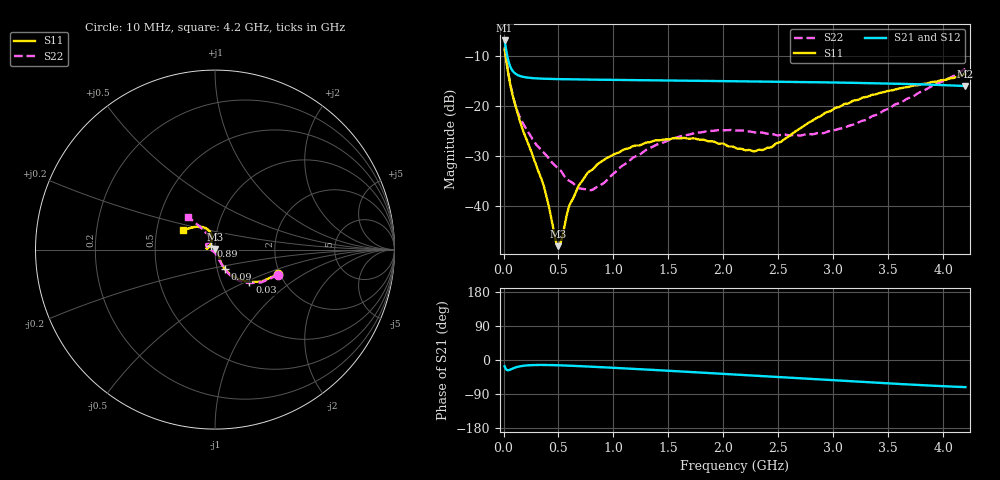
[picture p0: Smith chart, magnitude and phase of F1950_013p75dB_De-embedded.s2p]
! Integrated Device Technology
! Corporate Headquarters
! 6024 Silver Creek Valley Road
! San Jose, CA 95138  USA
! Phone:  1-408-284-8200
! Toll Free:  1-800-223-1366
! Webpage:  http://www.idt.com/
! Timing and RF Division
! 515 Groton Road, Suite 102
! Westford, MA 01886-6024
! Device:  F1950
! Description: 7-bit 0.25 dB Digital Step Attenuator
! Frequency:  150.0 -  4000.00 MHz
! Package:  4x4 mm Thin QFN Plastic Package: 24 pin
! Ports:  2 RF, 12 DC
!  Pin  1  = D0
!  Pin  2  = VDD
!  Pin  3  = Vmode
!  Pin  4  = GND
!  Pin  5  = RF1  =  Port 1
!  Pin  6  = GND
!  Pin  7  = GND
!  Pin  8  = GND
!  Pin  9  = GND
!  Pin 10  = GND
!  Pin 11  = GND
!  Pin 12  = GND
!  Pin 13  = GND
!  Pin 14  = RF2  =  Port 2
!  Pin 15  = GND
!  Pin 16  = LE
!  Pin 17  = CLK
!  Pin 18  = DATE
!  Pin 19  = D6
!  Pin 20  = D5
!  Pin 21  = D4
!  Pin 22  = D3
!  Pin 23  = D2
!  Pin 24  = D1
! State:  55
! Atten State:  13.75 dB
! Voltage:  +5.00 Volts
! Current:  Not Measured mA
! Data:  The device was measured on a the F195X evaluation board which has
!  individual transmission lines to the RF pins.  Data was collected
!  using a calibrated network analyzer.  The evaluation board was
!  de-embedded using a TRL calibration technique.
!  The reference plane is the edge of the package pin.
! Misc:  Board 2019
!  Action Tracker AT0250
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# GHz S dB R 50
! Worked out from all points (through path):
!   420 points, 10 MHz to 4.2 GHz, reference 50 ohm
!   highest |S21| = -6.84 dB at 10 MHz (marker M1); lowest = -16.0 dB at 4.2 GHz (marker M2)
!   group delay of S21, straight-line fit = 41.8 ps
!   lowest |S11| = -48.1 dB at 500 MHz (marker M3), VSWR 1.01, Z = 50.3 + j0.291 ohm
!   |S11| at or under -10 dB: 19.74 MHz to end of sweep
!   |S22| runs from -36.9 to -8.4 dB; largest |S21 - S12| = 0.00027
!   S11 on the Smith chart (normalised r, x): 10 MHz: 1.95, -0.62; 30 MHz: 1.36, -0.53; 90 MHz: 1.09, -0.24; 890 MHz: 0.96, +0.03; 4.2 GHz: 0.68, +0.16
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0.01  -8.48 -21.3  -6.84 -16.6  -6.84 -16.6  -8.43 -22.0
0.03  -11.57 -43.3  -9.50 -26.3  -9.50 -26.3  -11.48 -44.5
0.05  -14.36 -54.1  -11.37 -26.6  -11.37 -26.6  -14.15 -55.5
0.09  -18.46 -63.2  -13.13 -21.7  -13.13 -21.7  -18.36 -63.1
0.15  -23.07 -64.8  -13.97 -16.6  -13.97 -16.6  -22.30 -67.2
0.26  -29.59 -58.1  -14.39 -13.5  -14.39 -13.5  -26.50 -69.3
0.37  -36.35 -44.1  -14.52 -13.1  -14.52 -13.1  -29.41 -72.3
0.47  -46.48 3.9  -14.58 -13.7  -14.58 -13.7  -31.97 -78.7
0.5  -48.12 47.4  -14.60 -13.9  -14.60 -13.9  -32.50 -80.7
0.53  -46.66 79.3  -14.61 -14.2  -14.61 -14.2  -33.26 -81.7
0.6  -39.92 112.1  -14.64 -15.0  -14.64 -15.0  -35.03 -93.2
0.71  -35.20 126.1  -14.67 -16.4  -14.67 -16.4  -36.58 -113.4
0.89  -31.15 139.6  -14.72 -18.9  -14.72 -19.0  -35.75 -154.9
1.17  -28.12 154.5  -14.80 -23.2  -14.80 -23.2  -30.48 174.4
1.41  -26.87 165.7  -14.86 -27.0  -14.86 -27.0  -27.59 164.7
1.73  -26.49 173.2  -14.93 -32.1  -14.93 -32.1  -25.45 155.8
2.11  -28.39 163.8  -15.03 -38.5  -15.03 -38.5  -24.91 145.9
2.43  -28.31 127.5  -15.11 -43.7  -15.11 -43.8  -25.58 135.0
2.81  -22.93 104.3  -15.21 -50.2  -15.21 -50.3  -25.67 118.7
3.1  -19.58 106.8  -15.31 -55.2  -15.31 -55.2  -24.34 113.8
3.51  -16.91 118.4  -15.49 -61.9  -15.48 -61.9  -20.47 116.3
4.2  -13.58 148.4  -15.98 -71.6  -15.98 -71.7  -12.55 129.5
